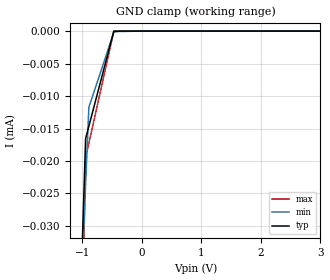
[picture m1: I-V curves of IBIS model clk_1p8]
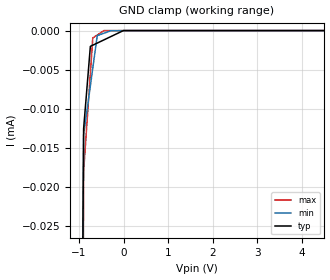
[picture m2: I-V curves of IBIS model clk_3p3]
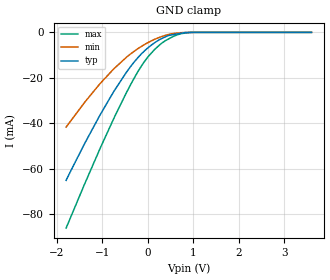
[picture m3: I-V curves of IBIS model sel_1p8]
|Texas Instruments Incorporated
|SDIO Port Expander With Voltage-Level Translation
|Marketing part#   Digital Voltage Range  Package-type   #pins
|TXS02612RTWR   1.1V - 3.6V   QFN   24
|TXS02612ZQSR   1.1V - 3.6V   MicroStar Junior BGA  24
[IBIS Ver]   3.2
[File name]   txs02612.ibs
[File Rev]   1.0
[Date]   6/18/2012
[Source]
| Texas Instruments Incorporated.
| Analog-eLab Design Center, HPA
| 12500 TI Blvd
| Dallas, TX -75243
| e-mail: elab_scm_ibis@list.ti.com
[Notes]   Revision History:
| Rev 1.0: 6/18/2012
| - Initial version of the model
| - Model generated from simulations in TISPICE
| - Model matched to SPICE simulation
| - C_comp although listed in numerical order of value are
|   obtained from varying PVT conditions. For PVT conditions for
|   each specific value refer the buffer description under
|   respective [Model]. IBIS model user is responsible for using
|   appropriate C_comp to simulate for Signal Integrity.
| - Model names with a trailing _1p8 contains the model for
|   1.8V [1.71V and 1.89V]. Model names with a trailing _3p3
|   contains the model for 3.3V [3.0V and 3.6V].
|*  EXCEPTION:   *
|*  - For model sel_*, there will be small leakage current in the GND   *
|*   clamp I-V Table because of a transistor named MN1 connected   *
|*   on the pad.   *
[Disclaimer]
| This model is designed as an aid for customers of Texas Instruments.
| TI and its licensors and suppliers make no warranties, either expressed
| or implied, with respect to this  model, including the warranties of
| merchantability or fitness for a particular purpose. The model is
| provided solely on an "as is" basis. The entire risk as to its quality
| and performance is with the customer.
[Copyright]
(C) Copyright 2012 Texas Instruments Incorporated.All rights reserved.
|   TXS02612RTW
[Component]   TXS02612RTW
[Manufacturer]   TI
[Package]   |24 QFN   -  RTW package
|   typ   min   max
R_pkg   0.05873   0.04341   0.09089
L_pkg   0.80209nH   0.58262nH   1.30592nH
C_pkg   0.28714pF   0.20076pF   0.49241pF
[Pin]  signal_name   model_name   R_pin   L_pin   C_pin
1   DAT2A   A_CMD   0.05620   0.83792nH  0.20815pF
2   GND   GND   0.04140   0.55885nH  0.21447pF
3   DAT3A   A_CMD   0.04341   0.58262nH  0.21025pF
4   CMDA   A_CMD   0.04376   0.60716nH  0.20976pF
5   VCCA   POWER   0.05624   0.78384nH  0.19930pF
6   DAT0A   A_CMD   0.05038   0.73180nH  0.22858pF
7   DAT1A   A_CMD   0.09089   1.30592nH  0.49241pF
8   DAT2B1   B_CMD   0.06614   0.85327nH  0.40297pF
9   CLKA   CLK   0.06559   0.89596nH  0.37699pF
10   DAT3B1   B_CMD   0.05289   0.75003nH  0.23042pF
11   GND   GND   0.04731   0.71545nH  0.21852pF
12   CMDB1   B_CMD   0.07443   0.92717nH  0.41275pF
13   CLKB1   CLKB   0.07624   0.95178nH  0.41604pF
14   DAT0B1   B_CMD   0.05305   0.74206nH  0.22057pF
15   DAT1B1   B_CMD   0.05097   0.70644nH  0.22694pF
16   DAT1B0   B_CMD   0.06526   0.83101nH  0.37381pF
17   VCCB1   POWER   0.06609   0.85168nH  0.41004pF
18   DAT0B0   B_CMD   0.07390   0.94932nH  0.38104pF
19   CLKB0   CLKB   0.05456   0.73330nH  0.21748pF
20   CMDB0   B_CMD   0.05572   0.82430nH  0.20550pF
21   VCCB0   POWER   0.04278   0.59438nH  0.20792pF
22   DAT3B0   B_CMD   0.04370   0.60111nH  0.21450pF
23   DAT2B0   B_CMD   0.04621   0.65024nH  0.22677pF
24   SEL   SEL   0.05252   0.75821nH  0.20076pF
|   TXS02612ZQS
[Component]   TXS02612ZQS
[Manufacturer]   TI
[Package]   |24 MicroStar Junior BGA -  ZQS package
|   typ   min   max
R_pkg   0.07876   0.05956   0.24323
L_pkg   1.28785nH   1.13325nH   1.44515nH
C_pkg   0.22775pF   0.13798pF   0.26115pF
[Pin]  signal_name   model_name   R_pin   L_pin   C_pin
A1   DAT2A   A_CMD   0.07784   1.42910nH  0.22699pF
A2   SEL   SEL   0.05956   1.13325nH  0.22743pF
A3   DAT3B0   B_CMD   0.06180   1.16223nH  0.23854pF
A4   CMDB0   B_CMD   0.06281   1.18153nH  0.23193pF
A5   CLKB0   CLKB   0.07451   1.33286nH  0.21615pF
B1   DAT3A   A_CMD   0.07182   1.31867nH  0.25270pF
B3   DAT2B0   B_CMD   0.07152   1.44515nH  0.26115pF
B4   VCCB0   POWER   0.07157   1.26565nH  0.13904pF
B5   DAT0B0   B_CMD   0.07367   1.33993nH  0.24998pF
C1   CMDA   A_CMD   0.07076   1.30307nH  0.24890pF
C2   VCCA   POWER   0.08134   1.59860nH  0.26997pF
C3   GND   GND   0.08980   2.01637nH  0.33866pF
C4   VCCB1   POWER   0.08436   1.63640nH  0.27778pF
C5   DAT1B0   B_CMD   0.07345   1.33754nH  0.25200pF
D1   DAT0A   A_CMD   0.07071   1.30184nH  0.24672pF
D2   CLKA   CLK   0.07008   1.24273nH  0.13798pF
D3   GND   GND   0.07061   1.42732nH  0.26233pF
D4   DAT1B1   B_CMD   0.08179   1.41881nH  0.15099pF
D5   DAT0B1   B_CMD   0.07355   1.34455nH  0.24323pF
E1   DAT1A   A_CMD   0.24323   1.36592nH  0.21914pF
E2   DAT2B1   B_CMD   0.06159   1.16413nH  0.23104pF
E3   DAT3B1   B_CMD   0.06242   1.17050nH  0.24034pF
E4   CMDB1   B_CMD   0.06524   1.21184nH  0.24077pF
E5   CLKB1   CLKB   0.07006   1.26551nH  0.21127pF
|   Model Selectors
[Model Selector] CLK
clk_1p8   1.8V  digital input
clk_3p3   3.3V  digital input
[Model Selector] SEL
sel_1p8   1.8V  digital input
sel_3p3   3.3V  digital input
[Model Selector] CLKB
clkb_1p8   1.8V  digital output
clkb_3p3   3.3V  digital output
[Model Selector] A_CMD
a_cmd_1p8   1.8V  digital I/O
a_cmd_3p3   3.3V  digital I/O
[Model Selector] B_CMD
b_cmd_1p8   1.8V  digital I/O
b_cmd_3p3   3.3V  digital I/O
| Models and submodels in the file (10): clk_1p8 (Input), clk_3p3 (Input), sel_1p8 (Input), sel_3p3 (Input), clkb_1p8 (Output), clkb_3p3 (Output), a_cmd_1p8 (I/O), a_cmd_3p3 (I/O), b_cmd_1p8 (I/O), b_cmd_3p3 (I/O)
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|   clk_1p8 Model
[Model]   clk_1p8
Model_type   Input
Vinl = 0.63
Vinh = 1.17
|   typ   min   max
|   (nom PVT)   (fast PVT)   (slow PVT)
|C_comp from frequency sweep method (F=60MHz)
|Average
|C_comp   1.847e-12   1.812e-12   1.849e-12
|C_comp from LC tank measurement(L=1nH)
|Average
|Resonant Frequency(Hz)   4.030e+09   4.040e+09   4.030e+09
C_comp   1.561e-12   1.553e-12   1.561e-12
[Model spec]
|subparameter
Vinl   0.63   0.599   0.662
Vinh   1.17   1.112   1.229
| Where nom  PVT is Nominal Process, 1.8V, 27C
|   Fast PVT is Strong Process,  1.89V, -40C
|   Slow PVT is Weak Process,   1.71V, 125C
[Voltage Range]   1.8   1.71   1.89
|Ambient Temperature   25   85   -40
|Junction Temperature
[Temperature Range]   27   125   -40
[Power Clamp Reference]   1.8   1.71   1.89
[GND Clamp Reference]   0   0   0
[GND Clamp]
|   Voltage   I(typ)   I(min)   I(max)
-1.8V     -915.9uA   -534.9uA   -1.388mA
-1.062V   -50.25uA   -49.12uA   -69.45uA
-945mV    -16.54uA   -23.55uA   -20.26uA
-941.2mV  -16.41uA   -22.73uA   -19.35uA
-890.9mV  -14.66uA   -11.75uA   -17.28uA
-470.6mV  -27.36nA   -162.4nA   0A
-68.4mV   0A         0A         0A
3.6V      0A         0A         0A
[POWER Clamp]
|   Voltage   I(typ)   I(min)   I(max)
-1.8V     0A         0A         0A
0V        0A         0A         0A
3.6V      0A         0A         0A
|   clk_3p3 Model
[Model]   clk_3p3
Model_type   Input
Vinl = 1.155
Vinh = 2.145
|   typ   min   max
|   (nom PVT)   (fast PVT)   (slow PVT)
|C_comp from frequency sweep method (F=60MHz)
|Average
|C_comp   1.722e-12   1.712e-12   1.785e-12
|C_comp from LC tank measurement(L=1nH)
|Average
|Resonant Frequency(Hz)   4.170e+09   4.170e+09   4.170e+09
C_comp   1.458e-12   1.458e-12   1.458e-12
[Model spec]
|subparameter
Vinl   1.155   1.05   1.26
Vinh   2.145   1.95   2.34
| Where nom  PVT is Nominal Process, 3.3V, 27C
|   Fast PVT is Strong Process,  3.6V, -40C
|   Slow PVT is Weak Process,   3V, 125C
[Voltage Range]   3.3   3   3.6
|Ambient Temperature   25   85   -40
|Junction Temperature
[Temperature Range]   27   125   -40
[Power Clamp Reference]   3.3   3   3.6
[GND Clamp Reference]   0   0   0
[GND Clamp]
|   Voltage   I(typ)   I(min)   I(max)
-3.3V     -9.139mA   -7.498mA   -11.44mA
-1.732V   -737.3uA   -706.8uA   -1.214mA
-897.6mV  -12.58uA   -13.85uA   -19.68uA
-897mV    -12.54uA   -13.35uA   -18.83uA
-896.4mV  -12.49uA   -13.33uA   -17.97uA
-745.8mV  -2.02uA    -7.074uA   -5.468uA
-691.2mV  -1.872uA   -4.807uA   -936.6nA
-591mV    -1.599uA   -647.5nA   -568nA
-439.2mV  -1.186uA   -338.6nA   0A
-285mV    -767.2nA   -24.77nA   0A
-3.3mV    0A         -10.3nA    0A
6.6V      0A         0A         0A
[POWER Clamp]
|   Voltage   I(typ)   I(min)   I(max)
-3.3V     0A         0A         0A
0V        0A         0A         0A
6.6V      0A         0A         0A
|   sel_1p8 Model
[Model]   sel_1p8
Model_type   Input
Vinl = 0.63
Vinh = 1.17
|   typ   min   max
|   (nom PVT)   (fast PVT)   (slow PVT)
|C_comp from frequency sweep method (F=60MHz)
|Average
|C_comp   2.921e-12   2.800e-12   3.408e-12
|C_comp from LC tank measurement(L=1nH)
|Average
|Resonant Frequency(Hz)   3.370e+09   3.430e+09   3.280e+09
C_comp   2.233e-12   2.155e-12   2.357e-12
[Model spec]
|subparameter
Vinl   0.63   0.599   0.662
Vinh   1.17   1.112   1.229
| Where nom  PVT is Nominal Process, 1.8V, 27C
|   Fast PVT is Strong Process,  1.89V, -40C
|   Slow PVT is Weak Process,   1.71V, 125C
[Voltage Range]   1.8   1.71   1.89
|Ambient Temperature   25   85   -40
|Junction Temperature
[Temperature Range]   27   125   -40
[Power Clamp Reference]   1.8   1.71   1.89
[GND Clamp Reference]   0   0   0
[GND Clamp]
|   Voltage   I(typ)   I(min)   I(max)
-1.8V     -65.1mA    -41.68mA   -86.12mA
-1.062V   -36.67mA   -22.77mA   -51.54mA
-748.8mV  -25.95mA   -16.03mA   -37.82mA
-470.3mV  -17.48mA   -10.91mA   -26.42mA
-230.6mV  -11.35mA   -7.298mA   -17.63mA
-90.72mV  -8.455mA   -5.541mA   -13.24mA
149.3mV   -4.554mA   -3.048mA   -7.506mA
275.9mV   -3.008mA   -2.013mA   -5.195mA
478.8mV   -1.252mA   -806.8uA   -2.635mA
655.8mV   -647.7uA   -260.6uA   -1.013mA
948.8mV   -10.86uA   -8.701uA   -33.96uA
3.6V      0A         0A         0A
[POWER Clamp]
|   Voltage   I(typ)   I(min)   I(max)
-1.8V     0A         0A         0A
0V        0A         0A         0A
3.6V      0A         0A         0A
